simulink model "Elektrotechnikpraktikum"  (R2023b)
settings: Solver=ode8  StartTime=0.0  StopTime=inf  FixedStep=0.0005  RelTol=1e-3  EnableMultiTasking=on
libraries: arduinolib x5, simulink x2, dspstat3 x1

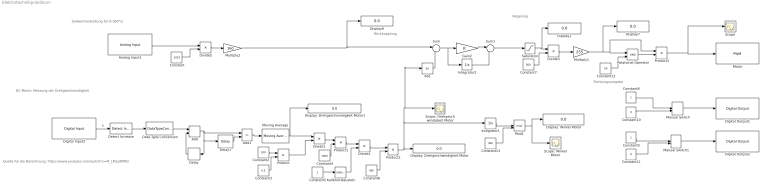
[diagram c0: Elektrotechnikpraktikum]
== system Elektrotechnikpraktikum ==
  note: Regelung
  note: Rückkopplung
  note: Sollwerteinstellung für 0-360°/s
  note: Richtungsvorgabe
  note: Quelle für die Berechnung: https://www.youtube.com/watch?v=M_LM1jdlPMQ
  note: DC-Motor: Messung der Drehgeschwindigkeit
  Abs : Abs
  Add : Sum
  Add1 : Sum  Inputs=+-
  Analog Input1 : arduinolib/Analog Input  pinNumber=0  ReadResultsOnly=off  ConversionTriggerSource=Software  ExternalTriggerType=uint32( 0 )  OutputDataType=uint16  EnableConversionCompleteNotify=off  EnableOuputStatus=off  SampleTime=-1  blockPlatform=arduino
  Constant : Constant  Value=1023
  Constant10 : Constant  Value=0
  Constant11 : Constant  Value=0
  Constant12 : Constant  Value=50
  Constant13 : Constant  Value=360
  Constant2 : Constant  Value=100
  Constant3 : Constant  Value=0.5
  Constant4 : Constant  Value=1000
  Constant5 : Constant
  Constant6 : Constant  Value=360
  Constant7 : Constant  Value=360
  Constant8 : Constant
  Constant9 : Constant
  Data Type Conversion : DataTypeConversion
  Delay : Delay  DelayLength=1
  Delay1 : Delay  DelayLength=100
  Detect Increase : simulink/Logic and Bit Operations/Detect Increase  vinit=0.0  OutDataTypeStr=boolean
  Digital Input2 : arduinolib/Digital Input  pinNumber=3  mode=Default  Direction=input  SampleTime=-1  blockPlatform=arduino
  Digital Output1 : arduinolib/Digital Output  pinNumber=10  Direction=output  blockPlatform=arduino
  Digital Output2 : arduinolib/Digital Output  pinNumber=9  Direction=output  blockPlatform=arduino
  Display1 : Display
  Display6 : Display
  Display7 : Display
  Display: Drehgeschwindigkeit Motor : Display
  Display: Drehgeschwindigkeit Motor1 : Display
  Display: Winkel Motor : Display
  Divide{1..3,5} (4 alike) : Product  Inputs=*/
  Gain2 : Gain
  Integrator1 : Integrator
  Integrator2 : Integrator
  Kalibrier-Baustein : simulink/Math Operations/Slider Gain  gain=494.0  low=0  high=950
  Manual Switch : ManualSwitch
  Manual Switch1 : ManualSwitch  CurrentSetting=0
  Mod1 : Math  Operator=mod
  Motor : arduinolib/PWM  pinNumber=11  frequencyType=Default  desiredFrequency=490.2  achievableFrequency=490.2
  Moving Average : dspstat3/Moving Average  Method=Sliding window  ForgettingFactorPort=off  SpecifyWindowLength=on  WindowLength=4  OverlapLength=3  AllowArbitraryInputLength=off  ForgettingFactor=0.9  SimulateUsing=Code generation
  Multiply1 : Gain  Gain=255
  Multiply2 : Gain  Gain=360
  Product{,1..3} (4 alike) : Product
  Relational Operator : RelationalOperator  OutDataTypeStr=boolean  RndMeth=Simplest
  Saturation : Saturate  UpperLimit=360  LowerLimit=0
  Scope : Scope
  Scope: Drehgeschwindigkeit Motor : Scope
  Scope: Winkel Motor : Scope
  Sum : Sum  Inputs=|+-
  Sum1 : Sum  Inputs=|++
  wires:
  Relational Operator/1 -> Product3/2
  Abs/1 -> Sum/2
  Divide3/1 -> Multiply1/1
  Constant12/1 -> Relational Operator/2
  Multiply1/1 -> Product3/1, Relational Operator/1, Display7/1
  Divide5/1 -> Multiply2/1
  Constant7/1 -> Divide3/2
  Constant/1 -> Divide5/2
  Analog Input1/1 -> Divide5/1
  Manual Switch1/1 -> Digital Output2/1
  Constant8/1 -> Manual Switch/1
  Constant11/1 -> Manual Switch1/2
  Manual Switch/1 -> Digital Output1/1
  Constant9/1 -> Manual Switch1/1
  Constant10/1 -> Manual Switch/2
  Constant2/1 -> Product/1
  Product2/1 -> Abs/1, Scope: Drehgeschwindigkeit Motor/1, Integrator1/1, Display: Drehgeschwindigkeit Motor/1
  Constant3/1 -> Product/2
  Constant5/1 -> Kalibrier-Baustein/1
  Constant13/1 -> Mod1/2
  Divide1/1 -> Product1/1
  Integrator1/1 -> Mod1/1
  Constant4/1 -> Product1/2
  Add/1 -> Delay/1, Delay1/1, Add1/1
  Divide2/1 -> Product2/1
  Delay1/1 -> Add1/2
  Delay/1 -> Add/2
  Constant6/1 -> Product2/2
  Data Type Conversion/1 -> Add/1
  Detect Increase/1 -> Data Type Conversion/1
  Product/1 -> Divide1/2
  Mod1/1 -> Scope: Winkel Motor/1, Display: Winkel Motor/1
  Digital Input2/1 -> Detect Increase/1  "6"
  Product1/1 -> Divide2/1
  Multiply2/1 -> Sum/1, Display6/1
  Moving Average/1 -> Display: Drehgeschwindigkeit Motor1/1, Divide1/1
  Product3/1 -> Scope/1, Motor/1
  Kalibrier-Baustein/1 -> Divide2/2
  Saturation/1 -> Display1/1, Divide3/1
  Sum/1 -> Integrator2/1, Gain2/1
  Add1/1 -> Moving Average/1
  Gain2/1 -> Sum1/1
  Sum1/1 -> Saturation/1
  Integrator2/1 -> Sum1/2
